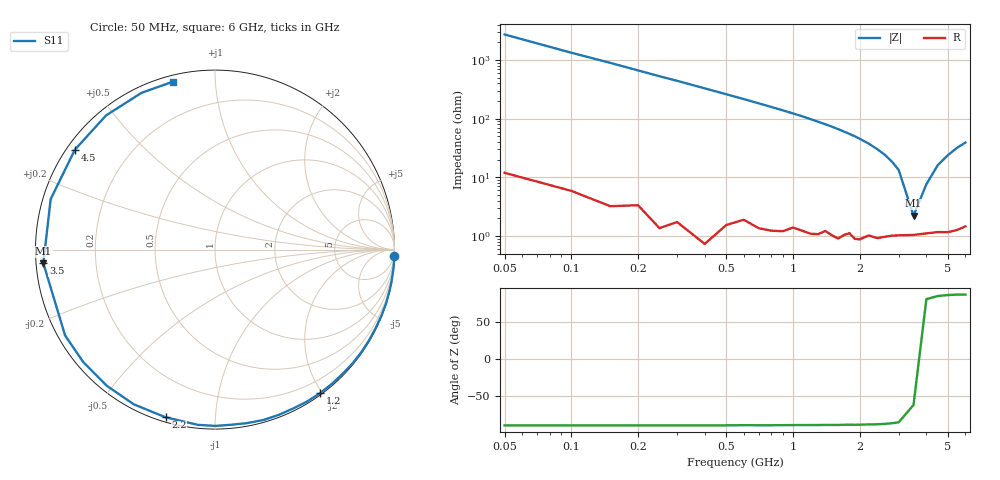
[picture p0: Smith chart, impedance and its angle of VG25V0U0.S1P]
! Infineon Technologies  Discrete & RF Semiconductors
! BB 831
! Si Tuning Diode in SOD323
! VR = 25 V
! S-Parameters:  July  1999
# GHz  S  MA  R  50
!  f  S11
! GHz  MAG  ANG
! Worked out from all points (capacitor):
!   34 points, 50 MHz to 6 GHz, reference 50 ohm
!   read as one part to ground: C = 1.18 pF near 50 MHz
!   lowest |Z| = 2.22 ohm at 3.5 GHz (marker M1)
!   series resonance near 3.604 GHz, so ESL is about 1.6 nH
!   S11 on the Smith chart (normalised r, x): 50 MHz: 0, -55; 1.2 GHz: 0.02, -1.97; 2.2 GHz: 0.02, -0.75; 3.5 GHz: 0.02, -0.04; 4.5 GHz: 0.02, +0.32; 6 GHz: 0.03, +0.78
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0.05  0.9998 -2.1
0.15  0.9996 -6.4
0.25  0.9995 -10.8
0.4  0.9993 -17.3
0.6  0.9962 -26.1
0.7  0.9962 -30.6
0.8  0.9956 -35.1
1  0.9921 -44.3
1.1  0.9916 -49.0
1.2  0.9911 -53.9
1.3  0.9897 -58.9
1.4  0.9865 -63.9
1.5  0.987 -68.8
1.6  0.987 -74.1
1.7  0.9832 -79.5
1.9  0.9823 -89.9
2  0.981 -95.5
2.2  0.9742 -106.4
2.4  0.9735 -117.7
2.6  0.9691 -128.5
2.8  0.9651 -139.6
3  0.9625 -150.2
3.5  0.9594 -175.5
4  0.9578 162.9
4.5  0.9586 144.5
5  0.9629 129.1
5.5  0.9647 115.1
6  0.9647 103.9
